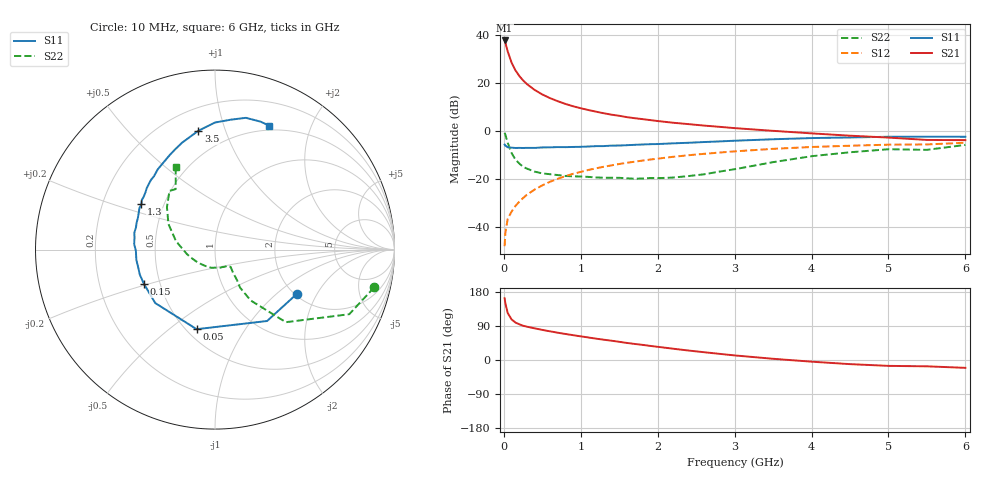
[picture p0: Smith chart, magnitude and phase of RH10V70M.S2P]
! SIEMENS Small Signal Semiconductors
! BFR106
! Si NPN RF Bipolar Junction Transistor in SOT23
! VCE = 10 V  IC = 70 mA
! Common Emitter S-Parameters:  August  1996
# GHz  S  MA  R  50
!  f  S11  S21  S12  S22
! GHz  MAG  ANG  MAG  ANG  MAG  ANG  MAG  ANG
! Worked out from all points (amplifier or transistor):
!   36 points, 10 MHz to 6 GHz, reference 50 ohm
!   highest |S21| = 37.8 dB at 10 MHz (marker M1)
!   |S21| within 3 dB of that: start of sweep to 36.98 MHz
!   unconditionally stable (mu >= 1): 228 MHz to 2.357 GHz
!   at 250 MHz: K = 1.02, MAG = 23.7 dB, |S12| = -28.1 dB
!   at 1.4 GHz: K = 1.07, MAG = 9.0 dB, |S12| = -14.4 dB
!   at 6 GHz: K = 0.98, MSG = 0.5 dB, |S12| = -4.9 dB
!   S11 on the Smith chart (normalised r, x): 10 MHz: 2.04, -1.38; 50 MHz: 0.56, -0.63; 150 MHz: 0.41, -0.19; 1.3 GHz: 0.37, +0.25; 3.5 GHz: 0.34, +0.81; 6 GHz: 0.45, +1.43
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0.01  0.5183 -28.5  77.63 162.9  0.0039 81.0  0.9111 -13.4
0.02  0.4924 -53.9  69.47 149.5  0.0075 70.5  0.8302 -25.7
0.05  0.4551 -103.0  45.92 124.1  0.0144 60.3  0.5651 -45.7
0.1  0.4467 -138.2  26.85 107.2  0.0205 61.3  0.3455 -55.0
0.15  0.4397 -154.3  18.51 98.9  0.0269 64.2  0.2534 -56.6
0.2  0.4414 -161.6  14.15 94.3  0.033 67.1  0.2087 -54.1
0.25  0.4394 -168.1  11.35 90.5  0.0395 69.2  0.1777 -52.8
0.3  0.442 -172.5  9.508 87.9  0.0464 70.5  0.1629 -52.0
0.4  0.4408 -179.1  7.193 83.6  0.0594 71.6  0.1409 -49.5
0.5  0.4514 176.1  5.774 79.4  0.0727 71.6  0.1294 -48.0
0.6  0.4533 171.7  4.841 75.7  0.0865 71.6  0.1245 -49.0
0.7  0.4592 168.1  4.179 72.0  0.0996 70.7  0.1195 -51.0
0.9  0.4618 161.1  3.276 65.5  0.1268 68.7  0.1123 -53.8
1.1  0.4718 154.3  2.728 59.4  0.1528 66.4  0.1093 -61.7
1.3  0.4816 148.4  2.335 53.5  0.1784 63.9  0.105 -69.0
1.6  0.5027 140.3  1.937 45.0  0.2156 60.1  0.1022 -84.0
2.2  0.5493 125.5  1.481 29.8  0.2873 51.8  0.1059 -120.8
2.8  0.6024 111.4  1.218 16.3  0.3524 43.2  0.1408 -161.3
3.5  0.6684 98.0  1.003 3.2  0.4217 33.2  0.2223 167.8
4.5  0.7298 82.9  0.794 -10.9  0.4898 18.6  0.3575 138.5
5.5  0.7567 70.4  0.647 -16.7  0.521 8.4  0.4022 123.0
6  0.7538 66.4  0.641 -20.7  0.5659 1.3  0.5098 115.4
